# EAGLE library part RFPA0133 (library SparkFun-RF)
IC PROG PWR AMP 16-QFN Source: Datasheet
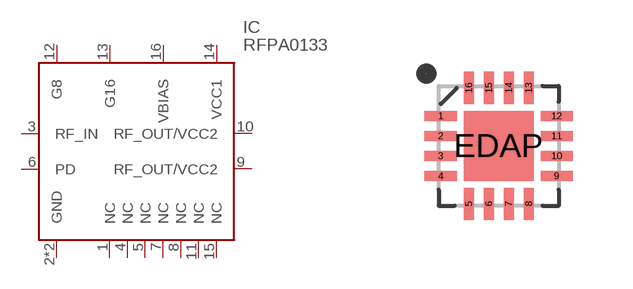
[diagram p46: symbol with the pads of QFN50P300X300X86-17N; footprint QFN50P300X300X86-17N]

Designator prefix IC

## RFPA0133 (MANUFACTURER_NAME: Qorvo; MANUFACTURER_PART_NUMBER: RFPA0133TR7; MOUSER_PART_NUMBER: 772-RFPA0133; PROD_ID: IC-15274)  [QFN50P300X300X86-17N]
1  NC  nc
2  GND  pwr
3  RF_IN  in
4  NC  nc
5  NC  nc
6  PD  in
7  NC  nc
8  NC  nc
9  RF_OUT/VCC2  out
10  RF_OUT/VCC2  out
11  NC  nc
12  G8  in
13  G16  in
14  VCC1  pwr
15  NC  nc
16  VBIAS  pwr
EDAP  GND  pwr

## Footprint QFN50P300X300X86-17N (pad centres in mm)
16-QFN
smd 0.8 x 0.25: 1 -1.45,0.75; 2 -1.45,0.25; 3 -1.45,-0.25; 4 -1.45,-0.75; 9 1.45,-0.75; 10 1.45,-0.25; 11 1.45,0.25; 12 1.45,0.75
smd 0.25 x 0.8: 5 -0.75,-1.45; 6 -0.25,-1.45; 7 0.25,-1.45; 8 0.75,-1.45; 13 0.75,1.45; 14 0.25,1.45; 15 -0.25,1.45; 16 -0.75,1.45
smd 1.75 x 1.75: EDAP 0,0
